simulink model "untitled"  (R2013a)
settings: Solver=ode23t  StartTime=0.0  StopTime=2  MaxStep=1e-3  RelTol=1e-4  AbsTol=1e-5
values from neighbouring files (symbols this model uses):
  m = v*BEAM.rho    [FlexBeamModelConstruct2.m]    (also in FlexBeamModelConstruct3.m = BEAM.rho*v; FlexBeam_1D_Construct.m = REF.m/REF.l*a.*(linspace(1-OPT.MassBiais+1e-6,1+OPT.MassBiai; FlexBeam_3D_Construct.m = REF.m/REF.l*a.*(linspace(1-OPT.MassBiais+1e-6,1+OPT.MassBiai; FreeFlexBeam_3D_Construct.m = REF.m/REF.l*a.*tmp2)
  N = D(1)+(H4^2+H3^2)/H2^2-(E(1)*H4+F(1)*H3)/H2    [MGD.m]    (also in MGD2.m)
  s = -sign(imag(KGZ_fr_tmp))    [LinprogReguliOptimFunc_1.m]    (also in LinprogReguliOptimFunc_2.m; LinprogReguliOptimFunc_1 - Copie.m)
  X = cos(phi(i))*x+sin(phi(i))*y    [MGI.m]
  Y = fft(y(:,i),NFFT)/L    [fft_bis.m]    (also in MGI.m = -sin(phi(i))*x+cos(phi(i))*y)
  Z = z    [MGI.m]
undefined symbols (not defined in the file or in its folder): deg, FLEX0, kg, rad
libraries: sm_lib x17, nesl_utility x3

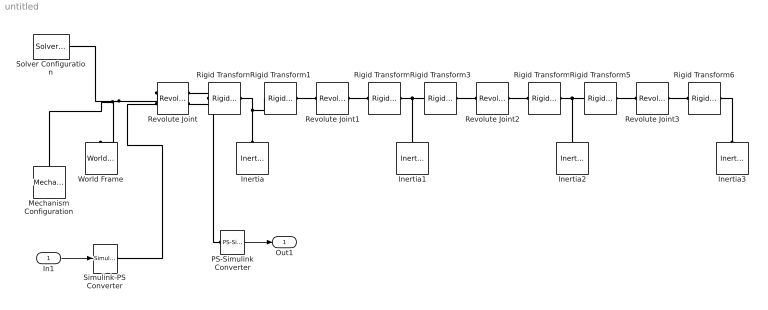
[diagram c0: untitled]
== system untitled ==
  In1 : Inport
  Inertia : sm_lib/Body Elements/Inertia  InertiaType=Custom  Mass=FLEX0.m(1)  MassUnits=kg  CenterOfMass=[0 0 0]  CenterOfMassUnits=m  MomentsOfInertia=[1 1 1].*FLEX0.J(1,2)  MomentsOfInertiaUnits=kg*m^2  ProductsOfInertia=[0 0 0]  ProductsOfInertiaUnits=kg*m^2  BlockFunction=simmechanics.library.body_elements.inertia
  Inertia1 : sm_lib/Body Elements/Inertia  InertiaType=Custom  Mass=FLEX0.m(2)  MassUnits=kg  CenterOfMass=[0 0 0]  CenterOfMassUnits=m  MomentsOfInertia=[1 1 1].*FLEX0.J(2,2)  MomentsOfInertiaUnits=kg*m^2  ProductsOfInertia=[0 0 0]  ProductsOfInertiaUnits=kg*m^2  BlockFunction=simmechanics.library.body_elements.inertia
  Inertia2 : sm_lib/Body Elements/Inertia  InertiaType=Custom  Mass=FLEX0.m(3)  MassUnits=kg  CenterOfMass=[0 0 0]  CenterOfMassUnits=m  MomentsOfInertia=[1 1 1].*FLEX0.J(3,2)  MomentsOfInertiaUnits=kg*m^2  ProductsOfInertia=[0 0 0]  ProductsOfInertiaUnits=kg*m^2  BlockFunction=simmechanics.library.body_elements.inertia
  Inertia3 : sm_lib/Body Elements/Inertia  InertiaType=Custom  Mass=FLEX0.m(4)  MassUnits=kg  CenterOfMass=[0 0 0]  CenterOfMassUnits=m  MomentsOfInertia=[1 1 1].*FLEX0.J(4,2)  MomentsOfInertiaUnits=kg*m^2  ProductsOfInertia=[0 0 0]  ProductsOfInertiaUnits=kg*m^2  BlockFunction=simmechanics.library.body_elements.inertia
  Mechanism Configuration : sm_lib/Utilities/Mechanism  Configuration  GravityVector=[0 0 -9.80665]  GravityUnits=m/s^2  AllowGravitySignal=off  LinearizationDelta=0.001  BlockFunction=simmechanics.library.utilities.mechanism_configuration
  PS-Simulink Converter : nesl_utility/PS-Simulink Converter  PhysicalDomain=network_engine_domain  SubClassName=ps_output  LeftPortType=input  RightPortType=output  PseudoPeriodic=off  Frequencies=[]  Unit=1  AffineConversion=off
  Revolute Joint : sm_lib/Joints/Revolute Joint  SenseConstraintForceX=off  SenseConstraintForceY=off  SenseConstraintForceZ=off  SenseConstraintTorqueX=off  SenseConstraintTorqueY=off  SenseConstraintTorqueZ=off  ConstraintWrenchDir=FollowerOnBase  ConstraintWrenchFrame=BaseFrame  EquilibriumPosition=0  EquilibriumPositionUnits=deg  SpringStiffness=FLEX0.k(1,5)  SpringStiffnessUnits=N*m/rad  DampingCoefficient=C  DampingCoefficientUnits=N*m/(deg/s)  ActuationMode=TorqueForceActuation  SensePosition=on  SenseVelocity=off  SenseAcceleration=off  SenseTorqueForce=off  PositionTargetValue=0  PositionTargetValueUnits=deg  PositionTargetSpecify=on  PositionTargetPriority=High  VelocityTargetValue=0  VelocityTargetValueUnits=deg/s  VelocityTargetSpecify=off  VelocityTargetPriority=High  BlockFunction=simmechanics.library.joints.revolute_joint
  Revolute Joint1 : sm_lib/Joints/Revolute Joint  SenseConstraintForceX=off  SenseConstraintForceY=off  SenseConstraintForceZ=off  SenseConstraintTorqueX=off  SenseConstraintTorqueY=off  SenseConstraintTorqueZ=off  ConstraintWrenchDir=FollowerOnBase  ConstraintWrenchFrame=BaseFrame  EquilibriumPosition=0  EquilibriumPositionUnits=deg  SpringStiffness=FLEX0.k(2,5)  SpringStiffnessUnits=N*m/rad  DampingCoefficient=C  DampingCoefficientUnits=N*m/(deg/s)  ActuationMode=NoActuation  SensePosition=off  SenseVelocity=off  SenseAcceleration=off  SenseTorqueForce=off  PositionTargetValue=0  PositionTargetValueUnits=deg  PositionTargetSpecify=on  PositionTargetPriority=High  VelocityTargetValue=0  VelocityTargetValueUnits=deg/s  VelocityTargetSpecify=off  VelocityTargetPriority=High  BlockFunction=simmechanics.library.joints.revolute_joint
  Revolute Joint2 : sm_lib/Joints/Revolute Joint  SenseConstraintForceX=off  SenseConstraintForceY=off  SenseConstraintForceZ=off  SenseConstraintTorqueX=off  SenseConstraintTorqueY=off  SenseConstraintTorqueZ=off  ConstraintWrenchDir=FollowerOnBase  ConstraintWrenchFrame=BaseFrame  EquilibriumPosition=0  EquilibriumPositionUnits=deg  SpringStiffness=FLEX0.k(3,5)  SpringStiffnessUnits=N*m/rad  DampingCoefficient=C  DampingCoefficientUnits=N*m/(deg/s)  ActuationMode=NoActuation  SensePosition=off  SenseVelocity=off  SenseAcceleration=off  SenseTorqueForce=off  PositionTargetValue=0  PositionTargetValueUnits=deg  PositionTargetSpecify=on  PositionTargetPriority=High  VelocityTargetValue=0  VelocityTargetValueUnits=deg/s  VelocityTargetSpecify=off  VelocityTargetPriority=High  BlockFunction=simmechanics.library.joints.revolute_joint
  Revolute Joint3 : sm_lib/Joints/Revolute Joint  SenseConstraintForceX=off  SenseConstraintForceY=off  SenseConstraintForceZ=off  SenseConstraintTorqueX=off  SenseConstraintTorqueY=off  SenseConstraintTorqueZ=off  ConstraintWrenchDir=FollowerOnBase  ConstraintWrenchFrame=BaseFrame  EquilibriumPosition=0  EquilibriumPositionUnits=deg  SpringStiffness=FLEX0.k(4,5)  SpringStiffnessUnits=N*m/rad  DampingCoefficient=C  DampingCoefficientUnits=N*m/(deg/s)  ActuationMode=NoActuation  SensePosition=off  SenseVelocity=off  SenseAcceleration=off  SenseTorqueForce=off  PositionTargetValue=0  PositionTargetValueUnits=deg  PositionTargetSpecify=on  PositionTargetPriority=High  VelocityTargetValue=0  VelocityTargetValueUnits=deg/s  VelocityTargetSpecify=off  VelocityTargetPriority=High  BlockFunction=simmechanics.library.joints.revolute_joint
  Rigid Transform : sm_lib/Frames and  Transforms/Rigid  Transform  TranslationMethod=Cartesian  TranslationLengthUnit=m  TranslationStandardAxis=+Z  TranslationStandardOffset=0  TranslationCartesianOffset=[FLEX0.b(1) 0 0]  TranslationROffset=0  TranslationROffsetUnits=m  TranslationZOffset=0  TranslationZOffsetUnits=m  TranslationThetaOffset=0  TranslationThetaOffsetUnits=deg  RotationMethod=None  RotationAngleUnits=deg  RotationStandardAxis=+Z  RotationAngle=0  RotationArbitraryAxis=[0 0 1]  FollAlignAxisA=+X  BaseAlignAxisA=+Y  FollAlignAxisB=+Y  BaseAlignAxisB=+Z  BlockFunction=simmechanics.library.frames_transforms.rigid_transform
  Rigid Transform1 : sm_lib/Frames and  Transforms/Rigid  Transform  TranslationMethod=Cartesian  TranslationLengthUnit=m  TranslationStandardAxis=+Z  TranslationStandardOffset=0  TranslationCartesianOffset=[FLEX0.a(1)-FLEX0.b(1) 0 0]  TranslationROffset=0  TranslationROffsetUnits=m  TranslationZOffset=0  TranslationZOffsetUnits=m  TranslationThetaOffset=0  TranslationThetaOffsetUnits=deg  RotationMethod=None  RotationAngleUnits=deg  RotationStandardAxis=+Z  RotationAngle=0  RotationArbitraryAxis=[0 0 1]  FollAlignAxisA=+X  BaseAlignAxisA=+Y  FollAlignAxisB=+Y  BaseAlignAxisB=+Z  BlockFunction=simmechanics.library.frames_transforms.rigid_transform
  Rigid Transform2 : sm_lib/Frames and  Transforms/Rigid  Transform  TranslationMethod=Cartesian  TranslationLengthUnit=m  TranslationStandardAxis=+Z  TranslationStandardOffset=0  TranslationCartesianOffset=[FLEX0.b(2) 0 0]  TranslationROffset=0  TranslationROffsetUnits=m  TranslationZOffset=0  TranslationZOffsetUnits=m  TranslationThetaOffset=0  TranslationThetaOffsetUnits=deg  RotationMethod=None  RotationAngleUnits=deg  RotationStandardAxis=+Z  RotationAngle=0  RotationArbitraryAxis=[0 0 1]  FollAlignAxisA=+X  BaseAlignAxisA=+Y  FollAlignAxisB=+Y  BaseAlignAxisB=+Z  BlockFunction=simmechanics.library.frames_transforms.rigid_transform
  Rigid Transform3 : sm_lib/Frames and  Transforms/Rigid  Transform  TranslationMethod=Cartesian  TranslationLengthUnit=m  TranslationStandardAxis=+Z  TranslationStandardOffset=0  TranslationCartesianOffset=[FLEX0.a(2)-FLEX0.b(2) 0 0]  TranslationROffset=0  TranslationROffsetUnits=m  TranslationZOffset=0  TranslationZOffsetUnits=m  TranslationThetaOffset=0  TranslationThetaOffsetUnits=deg  RotationMethod=None  RotationAngleUnits=deg  RotationStandardAxis=+Z  RotationAngle=0  RotationArbitraryAxis=[0 0 1]  FollAlignAxisA=+X  BaseAlignAxisA=+Y  FollAlignAxisB=+Y  BaseAlignAxisB=+Z  BlockFunction=simmechanics.library.frames_transforms.rigid_transform
  Rigid Transform4 : sm_lib/Frames and  Transforms/Rigid  Transform  TranslationMethod=Cartesian  TranslationLengthUnit=m  TranslationStandardAxis=+Z  TranslationStandardOffset=0  TranslationCartesianOffset=[FLEX0.b(3) 0 0]  TranslationROffset=0  TranslationROffsetUnits=m  TranslationZOffset=0  TranslationZOffsetUnits=m  TranslationThetaOffset=0  TranslationThetaOffsetUnits=deg  RotationMethod=None  RotationAngleUnits=deg  RotationStandardAxis=+Z  RotationAngle=0  RotationArbitraryAxis=[0 0 1]  FollAlignAxisA=+X  BaseAlignAxisA=+Y  FollAlignAxisB=+Y  BaseAlignAxisB=+Z  BlockFunction=simmechanics.library.frames_transforms.rigid_transform
  Rigid Transform5 : sm_lib/Frames and  Transforms/Rigid  Transform  TranslationMethod=Cartesian  TranslationLengthUnit=m  TranslationStandardAxis=+Z  TranslationStandardOffset=0  TranslationCartesianOffset=[FLEX0.a(3)-FLEX0.b(3) 0 0]  TranslationROffset=0  TranslationROffsetUnits=m  TranslationZOffset=0  TranslationZOffsetUnits=m  TranslationThetaOffset=0  TranslationThetaOffsetUnits=deg  RotationMethod=None  RotationAngleUnits=deg  RotationStandardAxis=+Z  RotationAngle=0  RotationArbitraryAxis=[0 0 1]  FollAlignAxisA=+X  BaseAlignAxisA=+Y  FollAlignAxisB=+Y  BaseAlignAxisB=+Z  BlockFunction=simmechanics.library.frames_transforms.rigid_transform
  Rigid Transform6 : sm_lib/Frames and  Transforms/Rigid  Transform  TranslationMethod=Cartesian  TranslationLengthUnit=m  TranslationStandardAxis=+Z  TranslationStandardOffset=0  TranslationCartesianOffset=[FLEX0.b(4) 0 0]  TranslationROffset=0  TranslationROffsetUnits=m  TranslationZOffset=0  TranslationZOffsetUnits=m  TranslationThetaOffset=0  TranslationThetaOffsetUnits=deg  RotationMethod=None  RotationAngleUnits=deg  RotationStandardAxis=+Z  RotationAngle=0  RotationArbitraryAxis=[0 0 1]  FollAlignAxisA=+X  BaseAlignAxisA=+Y  FollAlignAxisB=+Y  BaseAlignAxisB=+Z  BlockFunction=simmechanics.library.frames_transforms.rigid_transform
  Simulink-PS Converter : nesl_utility/Simulink-PS Converter  PhysicalDomain=network_engine_domain  SubClassName=ps_input  LeftPortType=input  RightPortType=output  PseudoPeriodic=off  Frequencies=[]  NoiseDistribution=none  NoiseParameters=[]  Unit=1  AffineConversion=off  InputFiltering=off  SimscapeFilterOrder=1  InputFilterTimeConstant=0.001  UdotUserProvided=1
  Solver Configuration : nesl_utility/Solver Configuration  PhysicalDomain=network_engine_domain  SubClassName=solver  LeftPortType=input  RightPortType=generic  Accelerate=off  Tones=[]  Harmonics=[]  SimulateNoise=off  Profile=off  UseLocalSampling=off  EnableSwitchedLinearOptims=on  FrequencyDomain=off  UseCCode=off  UseNewInitialization=off  DoDC=off  ResidualTolerance=1e-09  UseLocalSolver=off  LocalSolverChoice=NE_BACKWARD_EULER_ADVANCER  LocalSolverSampleTime=0.001  DoFixedCost=off  MaxNonlinIter=3  MaxModeIter=2  LinearAlgebra=Sparse  DelaysMemoryBudget=1024
  World Frame : sm_lib/Frames and  Transforms/World Frame  BlockFunction=simmechanics.library.frames_transforms.world_frame
  Out1 : Outport
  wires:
  PS-Simulink Converter/1 -> Out1/1
  In1/1 -> Simulink-PS Converter/1
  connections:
  Revolute Joint/LConn1 -- Solver Configuration/RConn1 -- Mechanism Configuration/RConn1 -- World Frame/RConn1
  Rigid Transform/LConn1 -- Revolute Joint/RConn1
  Inertia/RConn1 -- Rigid Transform1/LConn1 -- Rigid Transform/RConn1
  Rigid Transform2/RConn1 -- Rigid Transform3/LConn1 -- Inertia1/RConn1
  Rigid Transform2/LConn1 -- Revolute Joint1/RConn1
  Rigid Transform4/RConn1 -- Rigid Transform5/LConn1 -- Inertia2/RConn1
  Rigid Transform4/LConn1 -- Revolute Joint2/RConn1
  Inertia3/RConn1 -- Rigid Transform6/RConn1
  Rigid Transform6/LConn1 -- Revolute Joint3/RConn1
  Revolute Joint3/LConn1 -- Rigid Transform5/RConn1
  Revolute Joint2/LConn1 -- Rigid Transform3/RConn1
  Rigid Transform1/RConn1 -- Revolute Joint1/LConn1
  PS-Simulink Converter/LConn1 -- Revolute Joint/RConn2
  Simulink-PS Converter/RConn1 -- Revolute Joint/LConn2
